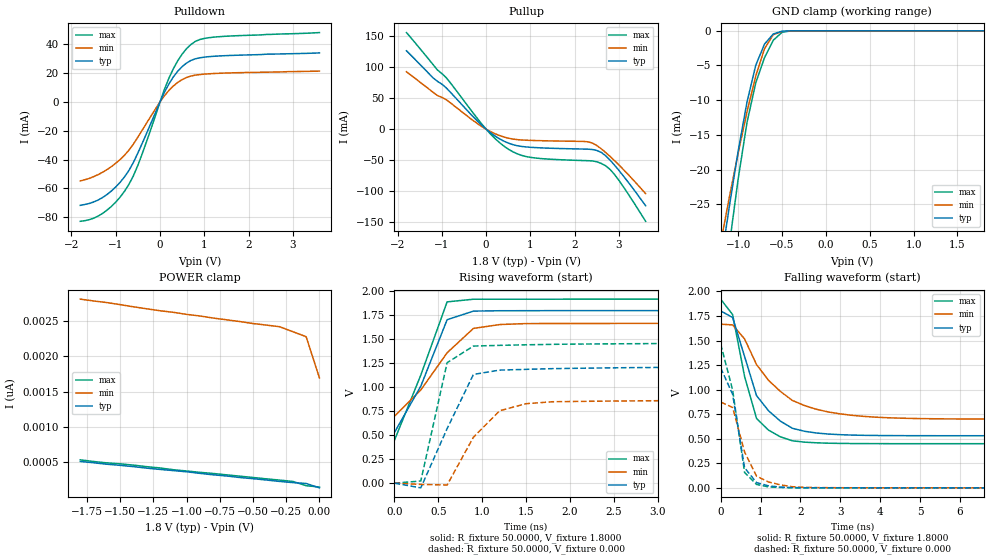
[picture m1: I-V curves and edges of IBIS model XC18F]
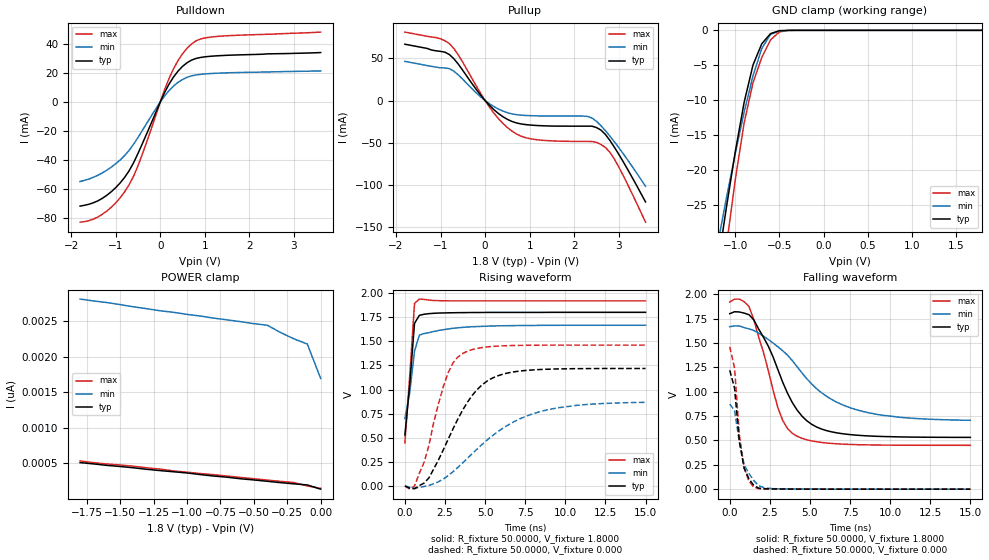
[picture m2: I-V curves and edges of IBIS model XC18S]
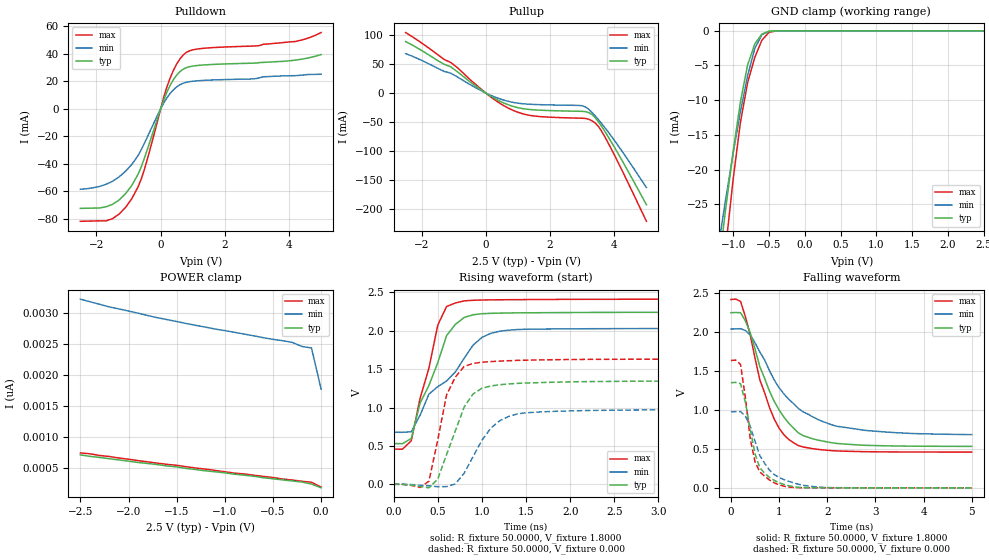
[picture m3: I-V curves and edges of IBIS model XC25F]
| Xilinx XC2CK IBIS File
[IBIS ver]   2.1
[File name]   xc2ck.ibs
[File Rev]   0.2
[Date]   Jul. 24, 2002
[Source]   Hspice simulations
[Notes]   Xilinx IBIS model for coolrunnerII
|   The available package models are
|   XC2C32  - CP56, VQ44 and PC44
|   XC2C64  - CP56, VQ44, VQ100 and PC44
|   XC2C128 - FT256, TQ144, CP132 and VQ100
|   XC2C256 - FT256, PQ208, TQ144, CP132, and VQ100
|   XC2C384 - FG324, FT256, PQ208, and TQ144
|   XC2C512 - FG324, FT256, and PQ208
|   with CP56 being selected as a default.
|   Please make your own selection of the packages by
|   commenting out the unused ones.
|   Control flag setting:
|   XC18F - 1.8V Vddio & fast slew rate
|   XC18S - 1.8V Vddio & slow slew rate
|   XC25F - 2.5V Vddio & fast slew rate
|   XC25S - 2.5V Vddio & slow slew rate
|   XC33F - 3.3V Vddio & fast slew rate
|   XC33S - 3.3V Vddio & slow slew rate
|   COMMENTS: Models include process corners for MIN and MAX
[Disclaimer]   The data in this model is derived from SPICE simulations
|   using modeling information extracted from the target pro-
|   cess. While a great deal of care has been take to provide
|   information that is accurate, this model is considered
|   preliminary as it has not been verified by actual silicon
|   measurement. Treat the data in this model as preliminary
|   until actual silicon verification is performed.
[Copyright]   Copyright 2002, Xilinx Inc., All rights reserved
[Component]   XC2Ck
[Manufacturer]   Xilinx Inc.
[Package]
|   Component XC2C32
|   >>> Make Your Selection of the Package type Below <<<
| For package type CP56
| variable   typ   min   max
R_pkg   89.0000m   75.0000m   103.000m
L_pkg   1.8500nH   1.5000nH   2.2000nH
C_pkg   0.3500pF   0.3000pF   0.4000pF
| For package type VQ44
| variable   typ   min   max
|R_pkg   57.0000m   54.0000m   60.0000m
|L_pkg   2.2500nH   2.1000nH   2.4000nH
|C_pkg   0.3000pF   0.3000pF   0.3000pF
| For package type PC44
| variable   typ   min   max
|R_pkg   67.5000m   66.0000m   69.0000m
|L_pkg   3.9500nH   3.6000nH   4.3000nH
|C_pkg   0.9000pF   0.8000pF   1.0000pF
|   Component XC2C64
|   >>> Make Your Selection of the Package type Below <<<
| For package type CP56
| variable   typ   min   max
|R_pkg   89.0000m   75.0000m   103.000m
|L_pkg   1.8500nH   1.5000nH   2.2000nH
|C_pkg   0.3500pF   0.3000pF   0.4000pF
| For package type VQ44
| variable   typ   min   max
|R_pkg   57.0000m   54.0000m   60.0000m
|L_pkg   2.2500nH   2.1000nH   2.4000nH
|C_pkg   0.3000pF   0.3000pF   0.3000pF
| For package type VQ100
| variable   typ   min   max
|R_pkg   119.500m   115.000m   124.000m
|L_pkg   6.1000nH   5.5000nH   6.7000nH
|C_pkg   0.6500pF   0.5000pF   0.8000pF
| For package type PC44
| variable   typ   min   max
|R_pkg   67.5000m   66.0000m   69.0000m
|L_pkg   3.9500nH   3.6000nH   4.3000nH
|C_pkg   0.9000pF   0.8000pF   1.0000pF
|   Component XC2C128
|   >>> Make Your Selection of the Package type Below <<<
| For package type FT256
| variable   typ   min   max
|R_pkg   188.500m   143.000m   234.000m
|L_pkg   4.9500nH   3.4000nH   6.5000nH
|C_pkg   0.7500pF   0.5000pF   1.0000pF
| For package type TQ144
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[Pin]  signal_name   model_name   R_pin   L_pin   C_pin
xc18f  xc18f   XC18F   NA   NA   NA
xc18s  xc18s   XC18S   NA   NA   NA
xc25f  xc25f   XC25F   NA   NA   NA
xc25s  xc25s   XC25S   NA   NA   NA
xc33f  xc33f   XC33F   NA   NA   NA
xc33s  xc33s   XC33S   NA   NA   NA
Vddio  vddio   POWER   NA   NA   NA
vgnd   gnd   GND   NA   NA   NA
| Models and submodels in the file (6): XC18F (I/O), XC18S (I/O), XC25F (I/O), XC25S (I/O), XC33F (I/O), XC33S (I/O)
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|   Model xc18f
[Model]   XC18F
Model_type   I/O
Polarity   Inverting
Enable   Active-High
Vinl =   0.8000V
Vinh =   1.2000V
Vmeas =   0.9000V
Cref =  50.0000pF
Rref =   1.0000M
Vref =  0.000V
C_comp   1.4810pF   0.9482pF   2.0140pF
[Temperature Range]   25.0000   100.0000   0.000
[Voltage Range]   1.8000V   1.7000V   1.9000V
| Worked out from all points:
|   slope of the pulldown table from 0 to 0.27 V, typ, clamps not added: 17 ohm
|   slope of the pullup table from 0 to 0.27 V, typ, clamps not added: 19.2 ohm
|   GND clamp passes 1 mA (typ) near -0.64 V on its own axis
|   rising waveform, R_fixture 50.0000, V_fixture 1.8000: 20-80 % time 373ps typ, 521ps min, 366ps max; typ from 0.529 V to 1.8 V
|   rising waveform, R_fixture 50.0000, V_fixture 0.000: 20-80 % time 374ps typ, 421ps min, 213ps max; typ from 0 V to 1.22 V
|   falling waveform, R_fixture 50.0000, V_fixture 1.8000: 20-80 % time 760ps typ, 1.14ns min, 509ps max; typ from 1.8 V to 0.531 V
|   falling waveform, R_fixture 50.0000, V_fixture 0.000: 20-80 % time 311ps typ, 453ps min, 363ps max; typ from 1.22 V to 0 V
[Pulldown]
| voltage   I(typ)   I(min)   I(max)
-1.8V     -71.81mA   -54.84mA   -82.9mA
-1.5V     -69.49mA   -51.9mA    -80.79mA
-1.2V     -64.37mA   -47.05mA   -75.24mA
-900mV    -55.8mA    -39.97mA   -66.09mA
-700mV    -47.49mA   -33.42mA   -57.13mA
-500mV    -35.5mA    -24.46mA   -44.05mA
200mV     12.46mA    7.971mA    16.42mA
400mV     21.32mA    13.55mA    28.59mA
700mV     28.84mA    18.01mA    39.96mA
900mV     30.67mA    19.03mA    43.37mA
1.2V      31.68mA    19.72mA    44.97mA
3.6V      34.07mA    21.42mA    48.19mA
[Pullup]
| voltage   I(typ)   I(min)   I(max)
-1.8V     126.5mA    92.72mA    155.9mA
-1.2V     82.9mA     59.67mA    104.3mA
-900mV    66.58mA    47.48mA    82.98mA
-100mV    6.43mA     4.382mA    8.532mA
400mV     -19.24mA   -12.54mA   -27.21mA
700mV     -26.56mA   -16.77mA   -39.61mA
1V        -29.13mA   -18mA      -45.38mA
2.3V      -32.17mA   -20.28mA   -50.76mA
2.6V      -37.49mA   -31.66mA   -55.22mA
2.8V      -50.07mA   -44.06mA   -64.97mA
2.9V      -58.11mA   -50.82mA   -73.19mA
3.6V      -123.4mA   -103.9mA   -148.5mA
[GND_clamp]
| voltage   I(typ)   I(min)   I(max)
-1.8V     -89.59mA   -75.16mA   -106.6mA
-1.2V     -33.66mA   -30.6mA    -40.86mA
-1.1V     -25.24mA   -23.93mA   -30.77mA
-1V       -17.32mA   -17.6mA    -21.32mA
-900mV    -10.29mA   -11.7mA    -13.23mA
-800mV    -4.969mA   -6.512mA   -7.511mA
-700mV    -1.912mA   -2.585mA   -3.865mA
-600mV    -461.7uA   -562.3uA   -1.358mA
-500mV    -51.62uA   -96uA      -215.1uA
-400mV    -3.51uA    -19.18uA   -14.57uA
1.8V      137pA      2.581nA    128pA
[POWER_clamp]
| voltage   I(typ)   I(min)   I(max)
-1.8V     511.2pA    2.813nA    534.3pA
-1.6V     472.1pA    2.764nA    491.2pA
-1.4V     437.8pA    2.704nA    459.6pA
-1.2V     398.2pA    2.648nA    419.2pA
-1.1V     381.9pA    2.626nA    394.1pA
-500mV    266.9pA    2.467nA    284.1pA
-300mV    228.4pA    2.422nA    246.9pA
-200mV    211.2pA    2.351nA    228pA
-100mV    199.2pA    2.28nA     167.7pA
0V        136.9pA    1.695nA    148.4pA
[Ramp]
| variable   typ   min   max
dV/dt_r   0.7314/0.2251n   0.5236/0.3151n   0.8760/0.2163n
dV/dt_f   0.7616/0.6554n   0.5549/1.2201n   0.8879/0.4297n
R_load = 50.0000
[Rising Waveform]
R_fixture = 50.0000
V_fixture = 1.8000
V_fixture_min = 1.6000
V_fixture_max = 2.0000
L_fixture = 0.000H
C_fixture = 0.000F
| time   V(typ)   V(min)   V(max)
0s        528.9mV    698.1mV    448mV
300ps     1.012V     971.7mV    1.127V
600ps     1.704V     1.359V     1.891V
900ps     1.794V     1.613V     1.918V
1.2ns     1.798V     1.654V     1.918V
1.5ns     1.798V     1.664V     1.918V
15ns      1.8V       1.666V     1.919V
[Rising Waveform]
R_fixture = 50.0000
V_fixture = 0.000
V_fixture_min = 0.000
V_fixture_max = 0.000
L_fixture = 0.000H
C_fixture = 0.000F
| time   V(typ)   V(min)   V(max)
0s        241.8uV    375.9uV    -430.5uV
300ps     -49.06mV   -13.17mV   22.73mV
600ps     568.3mV    -19.73mV   1.256V
900ps     1.133V     479.4mV    1.429V
1.2ns     1.179V     755.3mV    1.437V
1.5ns     1.187V     828.6mV    1.443V
1.8ns     1.194V     848.9mV    1.448V
3.3ns     1.208V     861.6mV    1.456V
5.1ns     1.215V     868.1mV    1.46V
15ns      1.219V     872.7mV    1.46V
[Falling Waveform]
R_fixture = 50.0000
V_fixture = 1.8000
V_fixture_min = 1.6000
V_fixture_max = 2.0000
L_fixture = 0.000H
C_fixture = 0.000F
| time   V(typ)   V(min)   V(max)
0s        1.802V     1.667V     1.921V
300ps     1.734V     1.659V     1.764V
600ps     1.337V     1.516V     1.134V
900ps     939mV      1.255V     706.5mV
1.2ns     785.3mV    1.095V     587.8mV
1.5ns     678.8mV    981.3mV    519.3mV
1.8ns     606.4mV    889.9mV    479.1mV
2.7ns     547.9mV    772.8mV    454.6mV
4.2ns     532.2mV    713.7mV    450mV
15ns      530.7mV    699.7mV    449.6mV
[Falling Waveform]
R_fixture = 50.0000
V_fixture = 0.000
V_fixture_min = 0.000
V_fixture_max = 0.000
L_fixture = 0.000H
C_fixture = 0.000F
| time   V(typ)   V(min)   V(max)
0s        1.222V     873.5mV    1.464V
300ps     952.8mV    818.5mV    997.1mV
600ps     204.3mV    365.3mV    156.7mV
900ps     53.62mV    118.7mV    35.18mV
1.2ns     20.62mV    60.07mV    9.518mV
1.5ns     7.583mV    30.46mV    3.674mV
1.8ns     2.583mV    11.45mV    1.12mV
2.1ns     1.476mV    5.16mV     758.5uV
15ns      632.4nV    -1.023uV   -6.446uV
|   Model XC18S
[Model]   XC18S
Model_type   I/O
Polarity   Inverting
Enable   Active-High
Vinl =   0.8000V
Vinh =   1.2000V
Vmeas =   0.9000V
Cref =  50.0000pF
Rref =   1.0000M
Vref =  0.000V
C_comp   1.4810pF   0.9482pF   2.0140pF
[Temperature Range]   25.0000   100.0000   0.000
[Voltage Range]   1.8000V   1.7000V   1.9000V
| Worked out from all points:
|   slope of the pulldown table from 0 to 0.27 V, typ, clamps not added: 17 ohm
|   slope of the pullup table from 0 to 0.27 V, typ, clamps not added: 19.2 ohm
|   GND clamp passes 1 mA (typ) near -0.64 V on its own axis
|   rising waveform, R_fixture 50.0000, V_fixture 1.8000: 20-80 % time 387ps typ, 517ps min, 366ps max; typ from 0.528 V to 1.8 V
|   rising waveform, R_fixture 50.0000, V_fixture 0.000: 20-80 % time 2.37ns typ, 3.97ns min, 1.41ns max; typ from 0 V to 1.22 V
|   falling waveform, R_fixture 50.0000, V_fixture 1.8000: 20-80 % time 2.19ns typ, 3.71ns min, 1.52ns max; typ from 1.8 V to 0.531 V
|   falling waveform, R_fixture 50.0000, V_fixture 0.000: 20-80 % time 533ps typ, 749ps min, 503ps max; typ from 1.22 V to 0 V
[Pulldown]
| voltage   I(typ)   I(min)   I(max)
-1.8V     -71.81mA   -54.84mA   -82.9mA
-1.5V     -69.49mA   -51.9mA    -80.79mA
-1.2V     -64.37mA   -47.05mA   -75.24mA
-900mV    -55.8mA    -39.97mA   -66.09mA
-700mV    -47.49mA   -33.42mA   -57.13mA
-500mV    -35.5mA    -24.46mA   -44.05mA
200mV     12.46mA    7.971mA    16.42mA
400mV     21.32mA    13.55mA    28.59mA
700mV     28.84mA    18.01mA    39.96mA
900mV     30.67mA    19.03mA    43.37mA
1.2V      31.68mA    19.72mA    44.97mA
3.6V      34.07mA    21.42mA    48.19mA
[Pullup]
| voltage   I(typ)   I(min)   I(max)
-1.8V     66.94mA    46.57mA    81.37mA
-800mV    54.63mA    37.88mA    67.67mA
-600mV    43.16mA    30.45mA    54.12mA
100mV     -5.813mA   -3.882mA   -7.913mA
400mV     -19.24mA   -12.54mA   -27.21mA
700mV     -26.56mA   -16.76mA   -39.61mA
1.2V      -29.77mA   -18.28mA   -46.8mA
2.3V      -30.48mA   -18.89mA   -48.58mA
2.5V      -32.14mA   -24.7mA    -49.78mA
2.7V      -40.33mA   -35.85mA   -55.79mA
3V        -63.89mA   -55.99mA   -79.02mA
3.6V      -120.5mA   -102mA     -144.6mA
[GND_clamp]
| voltage   I(typ)   I(min)   I(max)
-1.8V     -89.59mA   -75.16mA   -106.6mA
-1.2V     -33.66mA   -30.6mA    -40.86mA
-1.1V     -25.24mA   -23.93mA   -30.77mA
-1V       -17.32mA   -17.6mA    -21.32mA
-900mV    -10.29mA   -11.7mA    -13.23mA
-800mV    -4.969mA   -6.512mA   -7.511mA
-700mV    -1.912mA   -2.585mA   -3.865mA
-600mV    -461.7uA   -562.3uA   -1.358mA
-500mV    -51.62uA   -96uA      -215.1uA
-400mV    -3.51uA    -19.18uA   -14.57uA
1.8V      136.9pA    2.58nA     127.9pA
[POWER_clamp]
| voltage   I(typ)   I(min)   I(max)
-1.8V     510.8pA    2.813nA    534.1pA
-1.6V     471.9pA    2.764nA    491.1pA
-1.4V     437.7pA    2.704nA    459.6pA
-1.2V     398.1pA    2.648nA    419pA
-1.1V     381.7pA    2.626nA    394.1pA
-500mV    266.7pA    2.467nA    283.9pA
-400mV    248pA      2.445nA    264.5pA
-300mV    228.4pA    2.342nA    246.8pA
-200mV    211.8pA    2.253nA    230.2pA
-100mV    196.3pA    2.18nA     181.9pA
0V        136.9pA    1.695nA    148.3pA
[Ramp]
| variable   typ   min   max
dV/dt_r   0.7308/2.3529n   0.5201/3.9598n   0.8760/1.4753n
dV/dt_f   0.7612/2.1741n   0.5501/3.5805n   0.8879/1.5722n
R_load = 50.0000
[Rising Waveform]
R_fixture = 50.0000
V_fixture = 1.8000
V_fixture_min = 1.6000
V_fixture_max = 2.0000
L_fixture = 0.000H
C_fixture = 0.000F
| time   V(typ)   V(min)   V(max)
0s        528.5mV    697.9mV    447.7mV
300ps     1.047V     964.5mV    1.135V
600ps     1.686V     1.398V     1.892V
900ps     1.768V     1.563V     1.938V
1.5ns     1.786V     1.589V     1.927V
2.7ns     1.795V     1.628V     1.919V
4.2ns     1.798V     1.651V     1.919V
7.5ns     1.799V     1.664V     1.919V
15ns      1.8V       1.666V     1.919V
[Rising Waveform]
R_fixture = 50.0000
V_fixture = 0.000
V_fixture_min = 0.000
V_fixture_max = 0.000
L_fixture = 0.000H
C_fixture = 0.000F
| time   V(typ)   V(min)   V(max)
0s        381.3uV    473.5uV    -282.1uV
600ps     -29.45mV   -22.6mV    -480uV
1.5ns     84.59mV    5.931mV    421.2mV
2.1ns     272.2mV    43.94mV    855.5mV
2.7ns     485.3mV    107.1mV    1.175V
3.6ns     786.4mV    239mV      1.373V
4.8ns     1.046V     428.6mV    1.435V
6.3ns     1.167V     618.9mV    1.454V
9.6ns     1.214V     811.8mV    1.46V
15ns      1.218V     866.8mV    1.46V
[Falling Waveform]
R_fixture = 50.0000
V_fixture = 1.8000
V_fixture_min = 1.6000
V_fixture_max = 2.0000
L_fixture = 0.000H
C_fixture = 0.000F
| time   V(typ)   V(min)   V(max)
0s        1.8V       1.667V     1.92V
600ps     1.818V     1.675V     1.95V
1.2ns     1.79V      1.645V     1.875V
2.4ns     1.469V     1.536V     1.218V
3ns       1.228V     1.461V     837.9mV
3.6ns     984.9mV    1.375V     622.4mV
4.2ns     811.6mV    1.256V     542.9mV
5.4ns     639mV      1.034V     486.5mV
7.8ns     555.3mV    819.8mV    457.3mV
15ns      531.3mV    706.6mV    449.7mV
[Falling Waveform]
R_fixture = 50.0000
V_fixture = 0.000
V_fixture_min = 0.000
V_fixture_max = 0.000
L_fixture = 0.000H
C_fixture = 0.000F
| time   V(typ)   V(min)   V(max)
0s        1.22V      872.5mV    1.461V
300ps     1.038V     809.2mV    1.244V
600ps     489.4mV    487mV      558.7mV
900ps     213.7mV    250.2mV    219.9mV
1.2ns     105.5mV    160.2mV    81.68mV
1.5ns     38.41mV    87.36mV    20.59mV
1.8ns     10.65mV    37.39mV    5.277mV
2.1ns     5.456mV    17.14mV    2.957mV
2.7ns     2.646mV    5.59mV     1.821mV
15ns      1.316uV    13.31uV    587.1nV
|   Model XC25F
[Model]   XC25F
Model_type   I/O
Polarity   Inverting
Enable   Active-High
Vinl =   0.8000V
Vinh =   1.7000V
Vmeas =   0.9000V
Cref =  50.0000pF
Rref =   1.0000M
Vref =  0.000V
C_comp   1.4810pF   0.9482pF   2.0140pF
[Temperature Range]   25.0000   100.0000   0.000
[Voltage Range]   2.5000V   2.4000V   2.6000V
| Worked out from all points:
|   slope of the pulldown table from 0 to 0.375 V, typ, clamps not added: 18.5 ohm
|   slope of the pullup table from 0 to 0.375 V, typ, clamps not added: 30.5 ohm
|   GND clamp passes 1 mA (typ) near -0.64 V on its own axis
|   rising waveform, R_fixture 50.0000, V_fixture 1.8000: 20-80 % time 330ps typ, 552ps min, 240ps max; typ from 0.531 V to 2.24 V
|   rising waveform, R_fixture 50.0000, V_fixture 0.000: 20-80 % time 278ps typ, 328ps min, 207ps max; typ from 0 V to 1.35 V
|   falling waveform, R_fixture 50.0000, V_fixture 1.8000: 20-80 % time 700ps typ, 991ps min, 553ps max; typ from 2.24 V to 0.531 V
|   falling waveform, R_fixture 50.0000, V_fixture 0.000: 20-80 % time 289ps typ, 452ps min, 242ps max; typ from 1.35 V to 0 V
[Pulldown]
| voltage   I(typ)   I(min)   I(max)
-2.5V     -72.4mA    -58.5mA    -81.8mA
-1.5V     -69.49mA   -52.7mA    -79.89mA
-900mV    -55.79mA   -40.51mA   -65.46mA
-700mV    -47.49mA   -33.88mA   -56.62mA
-500mV    -35.5mA    -24.82mA   -43.63mA
100mV     6.708mA    4.397mA    8.665mA
300mV     17.31mA    11.32mA    22.64mA
500mV     24.55mA    15.99mA    32.62mA
800mV     29.99mA    19.33mA    41.08mA
1.3V      31.88mA    20.67mA    43.98mA
4.2V      35.47mA    24.16mA    49mA
5V        39.52mA    25.18mA    55.51mA
[Pullup]
| voltage   I(typ)   I(min)   I(max)
-2.5V     89.13mA    68.26mA    104.7mA
-1.3V     49.75mA    37.47mA    58.09mA
-1.1V     45.53mA    34.53mA    53.1mA
200mV     -6.998mA   -5.045mA   -8.713mA
800mV     -22.19mA   -15.55mA   -28.72mA
1.5V      -28.98mA   -19.66mA   -39.6mA
3V        -31.59mA   -21.91mA   -43.51mA
3.2V      -33.65mA   -27.97mA   -45.11mA
3.4V      -42.2mA    -39.2mA    -51.55mA
3.6V      -57.32mA   -52.35mA   -65.55mA
3.8V      -74.74mA   -66.61mA   -85.33mA
5V        -193.1mA   -163.4mA   -221.8mA
[GND_clamp]
| voltage   I(typ)   I(min)   I(max)
-2.5V     -159.3mA   -132.2mA   -186.8mA
-1.2V     -33.66mA   -30.6mA    -40.86mA
-1.1V     -25.24mA   -23.93mA   -30.77mA
-1V       -17.33mA   -17.6mA    -21.32mA
-900mV    -10.3mA    -11.71mA   -13.24mA
-800mV    -4.969mA   -6.517mA   -7.512mA
-700mV    -1.912mA   -2.587mA   -3.865mA
-600mV    -461.7uA   -562.4uA   -1.358mA
-500mV    -51.63uA   -96.01uA   -215.1uA
-400mV    -3.51uA    -19.18uA   -14.58uA
2.5V      187.5pA    2.732nA    179pA
[POWER_clamp]
| voltage   I(typ)   I(min)   I(max)
-2.5V     717.2pA    3.218nA    748.9pA
-2.4V     693.8pA    3.176nA    735.6pA
-2.3V     676.6pA    3.135nA    707.8pA
-2.2V     656pA      3.093nA    691.9pA
-1.7V     562.5pA    2.919nA    584.4pA
-1.5V     525pA      2.859nA    550.6pA
-1.4V     500.3pA    2.826nA    527.6pA
-1.1V     446.4pA    2.737nA    468pA
-300mV    299.1pA    2.523nA    314.5pA
-200mV    282.2pA    2.458nA    294.1pA
-100mV    249.3pA    2.434nA    278.4pA
0V        188.4pA    1.772nA    199.6pA
[Ramp]
| variable   typ   min   max
dV/dt_r   0.8076/0.2351n   0.5840/0.3186n   0.9780/0.1789n
dV/dt_f   0.9271/0.9717n   0.6180/1.3138n   1.1543/0.7265n
R_load = 50.0000
[Rising Waveform]
R_fixture = 50.0000
V_fixture = 1.8000
V_fixture_min = 1.6000
V_fixture_max = 2.0000
L_fixture = 0.000H
C_fixture = 0.000F
| time   V(typ)   V(min)   V(max)
0s        530.7mV    677.8mV    458.1mV
200ps     597.8mV    683.6mV    566.7mV
300ps     1.058V     899.7mV    1.12V
400ps     1.287V     1.174V     1.513V
500ps     1.583V     1.272V     2.073V
600ps     1.936V     1.345V     2.315V
700ps     2.083V     1.465V     2.361V
1ns       2.221V     1.913V     2.4V
1.3ns     2.231V     2.006V     2.404V
5ns       2.241V     2.031V     2.411V
[Rising Waveform]
R_fixture = 50.0000
V_fixture = 0.000
V_fixture_min = 0.000
V_fixture_max = 0.000
L_fixture = 0.000H
C_fixture = 0.000F
| time   V(typ)   V(min)   V(max)
0s        0V         0V         0V
300ps     -28.81mV   -12.85mV   -40.9mV
400ps     -46.25mV   -19.46mV   41.03mV
500ps     68.32mV    -30.99mV   576.7mV
600ps     388mV      -30.31mV   1.166V
800ps     1.009V     146.5mV    1.536V
900ps     1.176V     360.7mV    1.573V
1.2ns     1.296V     826.5mV    1.604V
1.5ns     1.319V     931.5mV    1.616V
5ns       1.346V     973.4mV    1.63V
[Falling Waveform]
R_fixture = 50.0000
V_fixture = 1.8000
V_fixture_min = 1.6000
V_fixture_max = 2.0000
L_fixture = 0.000H
C_fixture = 0.000F
| time   V(typ)   V(min)   V(max)
0s        2.242V     2.033V     2.411V
200ps     2.242V     2.038V     2.386V
400ps     1.987V     1.957V     1.959V
600ps     1.55V      1.739V     1.381V
900ps     1.106V     1.38V      879.3mV
1.1ns     905.6mV    1.202V     679.6mV
1.3ns     764.6mV    1.077V     576.8mV
1.5ns     667.8mV    972.7mV    522.5mV
2.2ns     567.8mV    787.9mV    472.4mV
5ns       531.1mV    682mV      458.2mV
[Falling Waveform]
R_fixture = 50.0000
V_fixture = 0.000
V_fixture_min = 0.000
V_fixture_max = 0.000
L_fixture = 0.000H
C_fixture = 0.000F
| time   V(typ)   V(min)   V(max)
0s        1.346V     973.8mV    1.63V
200ps     1.333V     977.2mV    1.579V
300ps     1.093V     919.2mV    1.152V
400ps     750.5mV    789.3mV    630.1mV
500ps     434mV      595mV      333.8mV
600ps     257.5mV    413.6mV    203.7mV
900ps     95.11mV    170.8mV    64.19mV
1.4ns     7.079mV    45.63mV    2.771mV
1.9ns     1.362mV    6.912mV    638.8uV
5ns       8.124uV    37.31uV    2.052uV
